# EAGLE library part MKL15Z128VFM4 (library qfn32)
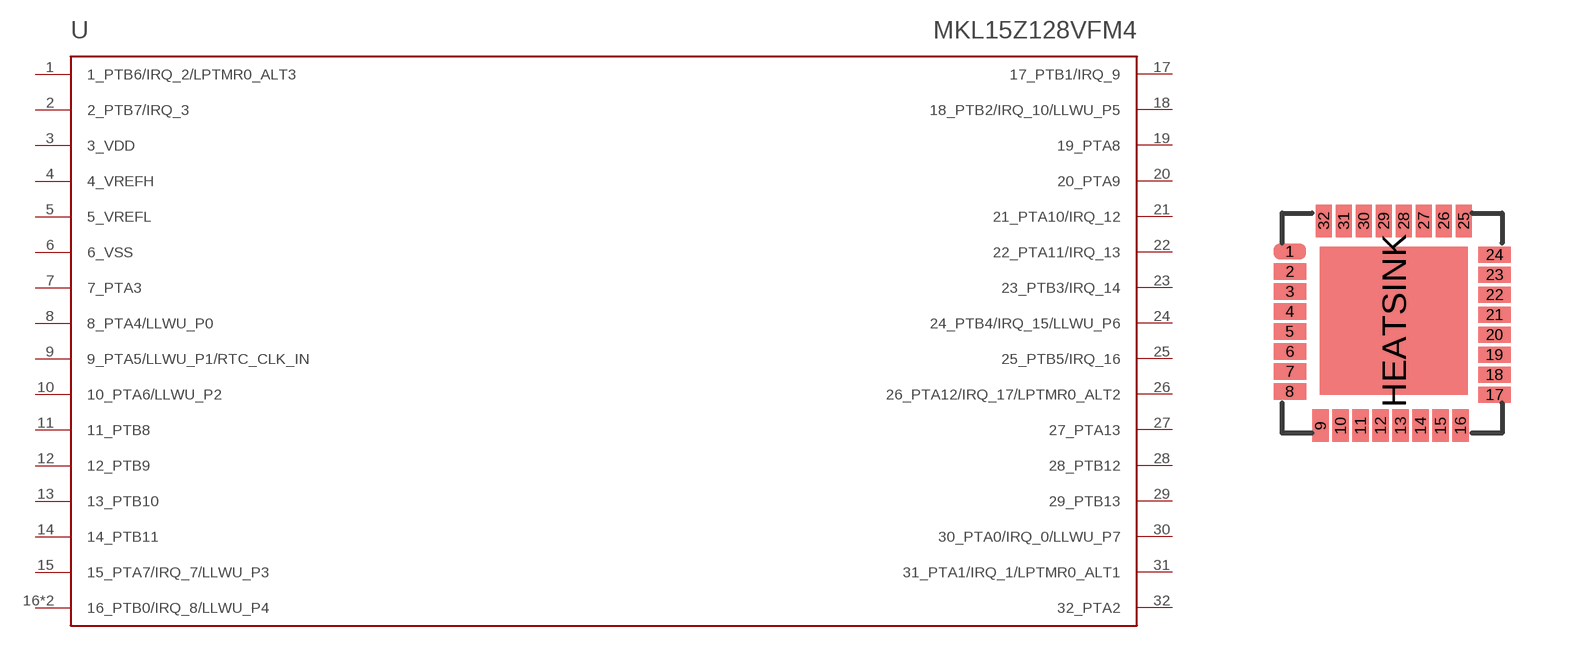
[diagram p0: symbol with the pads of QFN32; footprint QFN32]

Designator prefix -

## MKL15Z128VFM4  [QFN32]
1  1_PTB6/IRQ_2/LPTMR0_ALT3
2  2_PTB7/IRQ_3
3  3_VDD
4  4_VREFH
5  5_VREFL
6  6_VSS
7  7_PTA3
8  8_PTA4/LLWU_P0
9  9_PTA5/LLWU_P1/RTC_CLK_IN
10  10_PTA6/LLWU_P2
11  11_PTB8
12  12_PTB9
13  13_PTB10
14  14_PTB11
15  15_PTA7/IRQ_7/LLWU_P3
16  16_PTB0/IRQ_8/LLWU_P4
17  17_PTB1/IRQ_9
18  18_PTB2/IRQ_10/LLWU_P5
19  19_PTA8
20  20_PTA9
21  21_PTA10/IRQ_12
22  22_PTA11/IRQ_13
23  23_PTB3/IRQ_14
24  24_PTB4/IRQ_15/LLWU_P6
25  25_PTB5/IRQ_16
26  26_PTA12/IRQ_17/LPTMR0_ALT2
27  27_PTA13
28  28_PTB12
29  29_PTB13
30  30_PTA0/IRQ_0/LLWU_P7
31  31_PTA1/IRQ_1/LPTMR0_ALT1
32  32_PTA2
HEATSINK  16_PTB0/IRQ_8/LLWU_P4

## Footprint QFN32 (pad centres in mm)
smd 0.813 x 0.406: 1 -2.56,1.79; 2 -2.56,1.29; 3 -2.56,0.79; 4 -2.56,0.29; 5 -2.56,-0.21; 6 -2.56,-0.71; 7 -2.56,-1.21; 8 -2.56,-1.71; 17 2.56,-1.79; 18 2.56,-1.29; 19 2.56,-0.79; 20 2.56,-0.29; 21 2.56,0.21; 22 2.56,0.71; 23 2.56,1.21; 24 2.56,1.71
smd 0.406 x 0.813: 9 -1.79,-2.56; 10 -1.29,-2.56; 11 -0.79,-2.56; 12 -0.29,-2.56; 13 0.21,-2.56; 14 0.71,-2.56; 15 1.21,-2.56; 16 1.71,-2.56; 25 1.79,2.56; 26 1.29,2.56; 27 0.79,2.56; 28 0.29,2.56; 29 -0.21,2.56; 30 -0.71,2.56; 31 -1.21,2.56; 32 -1.71,2.56
smd 3.7 x 3.7: HEATSINK 0.04,0.06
